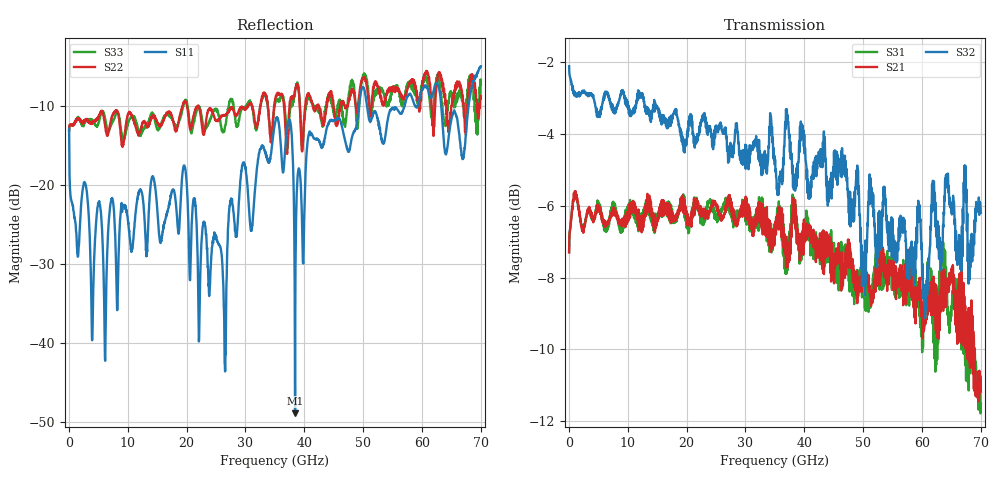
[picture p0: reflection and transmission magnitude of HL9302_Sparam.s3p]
! 2/22/2024 12:53:08 PM
! H:\PRODUCTION_DATA\TEMP_S3P.S3P
! CHANNEL.1
! TR.MEASUREMENT
! CORRECTED.DATA
# GHZ S RI R 50.0
! FREQ.GHZ  S11RE  S11IM  S12RE  S12IM  S13RE  S13IM
!  S21RE  S21IM  S22RE  S22IM  S23RE  S23IM
!  S31RE  S31IM  S32RE  S32IM  S33RE  S33IM
!; PortSelection: Port_123
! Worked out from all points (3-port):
!   2000 points, 35 MHz to 70 GHz, reference 50 ohm
!   strongest paths, dB at 35 MHz, 17.54 GHz, 35.03 GHz, 52.53 GHz, 70 GHz:
!     S32: -2.1, -3.5, -4.7, -7.3, -6.2
!     S21: -7.3, -6.4, -6.8, -8.2, -11.2
!     S31: -7.3, -6.1, -6.5, -7.7, -11.5
!   lowest |S11| = -48.9 dB at 38.43 GHz (marker M1), VSWR 1.01, Z = 49.6 - j0.0261 ohm
!   |S11| at or under -10 dB: start of sweep to 49.3 GHz; 50.64 GHz to 57.05 GHz (6.418 GHz wide, 11.9 % of centre); 63.26 GHz to 67.91 GHz (4.644 GHz wide, 7.08 % of centre)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
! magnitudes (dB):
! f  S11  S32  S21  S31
! 35 MHz  -12.9  -2.1  -7.3  -7.3
! 3.955 GHz  -39.7  -2.9  -6.3  -6.4
! 19.6 GHz  -17.6  -4.2  -6.2  -5.7
! 26.46 GHz  -42.6  -3.9  -6.2  -5.9
! 27.48 GHz  -22.1  -4.3  -5.8  -6.3
! 35.03 GHz  -12.1  -4.7  -6.8  -6.5
! 37.59 GHz  -12.0  -4.3  -6.8  -7.0
! 38.43 GHz  -48.9  -5.6  -5.8  -6.6
! 40.98 GHz  -13.4  -5.4  -6.9  -6.7
! 70 GHz  -5.0  -6.2  -11.2  -11.5
